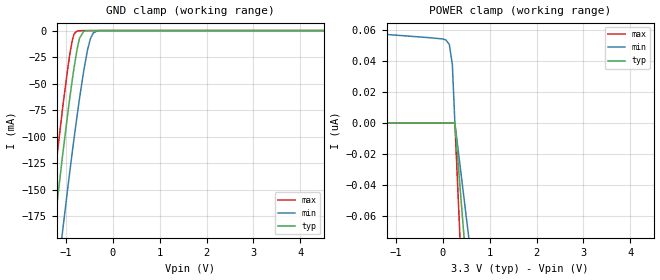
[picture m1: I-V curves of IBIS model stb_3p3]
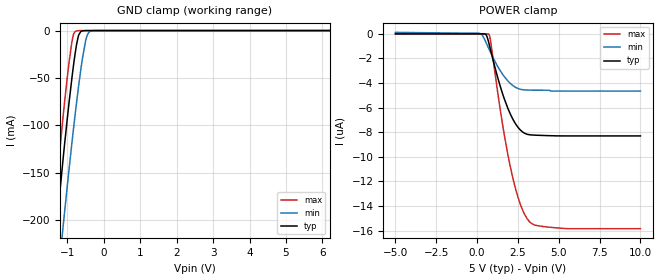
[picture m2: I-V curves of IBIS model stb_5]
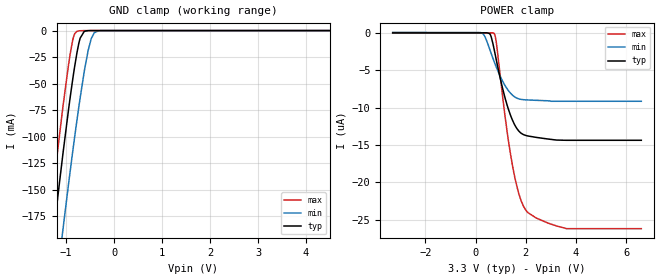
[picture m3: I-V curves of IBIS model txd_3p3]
|Texas Instruments Incorporated
|TCAN1042HGV-Q1 Automotive Fault Protected CAN Transceiver With Flexible
|Data-Rate
|Marketing part#   Digital Voltage Range   Package-type   #pins
|TCAN1042HGVDQ1   3-5.5V   SOIC   8
|TCAN1042HGVDRQ1   3-5.5V   SOIC   8
[IBIS Ver]   4.1
[File name]   tcan1042hgv_q1.ibs
[File Rev]   1.1
[Date]   4/13/2016
[Source]
| Texas Instruments Incorporated.
| Analog-eLab Design Center, HPA
| 12500 TI Blvd
| Dallas, TX -75243
[Notes]   Revision History:
| Rev 1.1: 04/13/2016
| -Second version of the model. Fine tuning canh_os and canl_od models.
| Rev 1.0: 3/31/2016
| - Initial version of the model
| - Model generated from simulations in SPECTRE
| - Model matched to SPICE simulation
| - C_comp although listed in numerical order of value are
|   obtained from varying PVT conditions. For PVT conditions for
|   each specific value refer the buffer description under
|   respective [Model]. IBIS model user is responsible for using
|   appropriate C_comp to simulate for Signal Integrity.
|* EXCEPTION:   *
|* - For models rxd_* pullup and pulldown IV tables does not pass through *
|*   zero because of resistors R6, R8, R14 connected to pad.   *
|* - For canh_os model pullup table does not pass through zero due to   *
|*   resistor network connected to PAD. Power clamp table has leakage due *
|*   to resistor network connected to PAD   *
|* - For canl_od model pulldown table does not pass through zero due to   *
|*   resistor network connected to PAD. Power clamp table has leakage due *
|*   to resistor network connected to PAD   *
|* - canh_os and canl_od VT irregularity not indicitive of silicon   *
|*   actual device shows smooth transition between dominant and recessive *
[Disclaimer]
| This model is designed as an aid for customers of Texas Instruments.
| TI and its licensors and suppliers make no warranties, either expressed
| or implied, with respect to this  model, including the warranties of
| merchantability or fitness for a particular purpose. The model is
| provided solely on an "as is" basis. The entire risk as to its quality
| and performance is with the customer.
[Copyright]
(C) Copyright 2016 Texas Instruments Incorporated.All rights reserved.
|   TCAN1042HGV_Q1D
[Component]   TCAN1042HGV_Q1D
[Manufacturer]   TI
[Package]   |8 SOIC - D Package
|   typ   min   max
R_pkg   0.068   0.038   0.098
L_pkg   2.235nH   1.713nH   2.756nH
C_pkg   0.393pF   0.337pF   0.449pF
[Pin]  signal_name   model_name   R_pin   L_pin   C_pin
1   TXD   txd   0.093   2.653n   0.337p
2   GND   gnd   0.038   1.716n   0.449p
3   VCC   power   0.038   1.713n   0.449p
4   RXD   rxd   0.093   2.657n   0.337p
5   VIO   power   0.098   2.756n   0.341p
6   CANL   canl_od   0.092   2.624n   0.363p
7   CANH   canh_os   0.075   2.301n   0.349p
8   STB   stb   0.094   2.677n   0.338p
[Diff_pin]   inv_pin   vdiff   tdelay_typ   tdelay_min   tdelay_max
7   6   NA   NA   NA   NA
|   Model Selectors
[Model Selector] stb
stb_3p3   3.3V   digital Input
stb_5   5.0V   digital Input
[Model Selector] txd
txd_3p3   3.3V   digital Input
txd_5   5.0V   digital Input
[Model Selector] rxd
rxd_3p3   3.3V   digital Output
rxd_5   5.0V   digital Output
| Models and submodels in the file (8): stb_3p3 (Input), stb_5 (Input), txd_3p3 (Input), txd_5 (Input), rxd_3p3 (Output), rxd_5 (Output), canh_os (I/O_open_source), canl_od (I/O_open_drain)
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|   stb_3p3 Model
[Model]   stb_3p3
Model_type   Input
Vinl = 0.99
Vinh = 2.31
|   typ   min   max
|   (nom PVT)   (fast PVT)   (slow PVT)
C_comp   2.287e-12   2.118e-12   2.744e-12
| Where nom  PVT is Nominal Process, 3.3V, 27C
|   Fast PVT is Strong Process,  3.6V, -55C
|   Slow PVT is Weak Process,   3V, 150C
[Voltage Range]   3.3   3   3.6
|Junction Temperature
[Temperature Range]   27   150   -55
[Power Clamp Reference]   3.3   3   3.6
[GND Clamp Reference]   0   0   0
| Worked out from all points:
|   GND clamp passes 1 mA (typ) near -0.62 V on its own axis
[GND Clamp]
|   Voltage   I(typ)   I(min)   I(max)
-3.3V     -1.097A    -1.144A    -1.073A
-1.386V   -241.5mA   -312mA     -198.2mA
-1.234V   -180.4mA   -251.7mA   -136mA
-1.066V   -115.8mA   -187.2mA   -71.51mA
-950.4mV  -74.68mA   -144.9mA   -32.42mA
-866.4mV  -47.18mA   -115.3mA   -9.84mA
-772.2mV  -20.38mA   -83.74mA   -682.4uA
-708mV    -7.173mA   -63.48mA   -166.8uA
-540mV    -73.56uA   -18.53mA   -2.625uA
-475.2mV  -13.82uA   -7.402mA   -445.1nA
-330mV    -246.1nA   -260uA     -18.22nA
6.6V      0A         0A         0A
[POWER Clamp]
|   Voltage   I(typ)   I(min)   I(max)
-3.3V     0A         61.82nA    0A
-330mV    0A         55.05nA    0A
-3mV      0A         54.15nA    0A
-2.4mV    0A         54.14nA    0A
0V        0A         54.13nA    0A
1.2mV     0A         54.12nA    0A
3mV       0A         54.11nA    0A
66mV      0A         53.48nA    0A
138mV     0A         50.7nA     0A
204mV     0A         37.79nA    0A
258mV     0A         0A         0A
6.6V      -2.384uA   -1.58uA    -4.306uA
|   stb_5 Model
[Model]   stb_5
Model_type   Input
Vinl = 1.5
Vinh = 3.5
|   typ   min   max
|   (nom PVT)   (fast PVT)   (slow PVT)
C_comp   2.287e-12   2.118e-12   2.744e-12
| Where nom  PVT is Nominal Process, 5V, 27C
|   Fast PVT is Strong Process,  5.5V, -55C
|   Slow PVT is Weak Process,   4.5V, 150C
[Voltage Range]   5   4.5   5.5
|Junction Temperature
[Temperature Range]   27   150   -55
[Power Clamp Reference]   5   4.5   5.5
[GND Clamp Reference]   0   0   0
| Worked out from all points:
|   GND clamp passes 1 mA (typ) near -0.63 V on its own axis
[GND Clamp]
|   Voltage   I(typ)   I(min)   I(max)
-5V       -1.891A    -1.922A    -1.879A
-1.522V   -297.1mA   -366.4mA   -255mA
-1.373V   -235.5mA   -306.2mA   -192mA
-1.115V   -133.6mA   -205.2mA   -88.9mA
-960mV    -77.39mA   -147.8mA   -34.81mA
-875mV    -49.33mA   -117.7mA   -11.28mA
-825.5mV  -34.35mA   -100.8mA   -3.153mA
-750mV    -14.76mA   -76.12mA   -386.7uA
-630mV    -838.1uA   -40.3mA    -25.63uA
-500mV    -25uA      -10.78mA   -774.5nA
-329mV    -233.3nA   -243.6uA   -34.68nA
10V       0A         0A         0A
[POWER Clamp]
|   Voltage   I(typ)   I(min)   I(max)
-5V       0A         120.9nA    0A
152.5mV   0A         51.48nA    0A
530.5mV   -35.11nA   -651.8nA   0A
725.5mV   -775.6nA   -1.229uA   -37.31nA
863mV     -1.51uA    -1.624uA   -924.4nA
1.6V      -5.031uA   -3.361uA   -7.707uA
2.11V     -6.734uA   -4.12uA    -11.27uA
2.407V    -7.425uA   -4.386uA   -12.86uA
2.772V    -7.967uA   -4.541uA   -14.29uA
3.344V    -8.225uA   -4.576uA   -15.43uA
5.505V    -8.303uA   -4.653uA   -15.85uA
10V       -8.303uA   -4.653uA   -15.85uA
|   txd_3p3 Model
[Model]   txd_3p3
Model_type   Input
Vinl = 0.99
Vinh = 2.31
|   typ   min   max
|   (nom PVT)   (fast PVT)   (slow PVT)
C_comp   2.287e-12   2.118e-12   2.744e-12
| Where nom  PVT is Nominal Process, 3.3V, 27C
|   Fast PVT is Strong Process,  3.6V, -55C
|   Slow PVT is Weak Process,   3V, 150C
[Voltage Range]   3.3   3   3.6
|Junction Temperature
[Temperature Range]   27   150   -55
[Power Clamp Reference]   3.3   3   3.6
[GND Clamp Reference]   0   0   0
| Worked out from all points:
|   GND clamp passes 1 mA (typ) near -0.62 V on its own axis
[GND Clamp]
|   Voltage   I(typ)   I(min)   I(max)
-3.3V     -1.097A    -1.144A    -1.073A
-1.386V   -241.5mA   -312mA     -198.2mA
-1.234V   -180.4mA   -251.7mA   -136mA
-1.066V   -115.8mA   -187.2mA   -71.49mA
-950.4mV  -74.68mA   -144.8mA   -32.4mA
-866.4mV  -47.17mA   -115.3mA   -9.833mA
-772.2mV  -20.38mA   -83.73mA   -677.4uA
-708mV    -7.169mA   -63.47mA   -163.5uA
-540mV    -73.3uA    -18.53mA   -2.704uA
-475.2mV  -13.88uA   -7.4mA     -723.7nA
-330mV    -361.7nA   -259.8uA   -278.1nA
6.6V      0A         0A         0A
[POWER Clamp]
|   Voltage   I(typ)   I(min)   I(max)
-3.3V     0A         61.83nA    0A
198mV     0A         38.13nA    0A
375mV     0A         -528.7nA   0A
558mV     -98.16nA   -2.148uA   0A
735.6mV   -2.148uA   -3.81uA    -62.66nA
831mV     -3.708uA   -4.639uA   -1.439uA
1.179V    -8.775uA   -7.084uA   -11.3uA
1.449V    -11.53uA   -8.275uA   -17.37uA
1.722V    -13.15uA   -8.838uA   -21.53uA
1.996V    -13.73uA   -8.968uA   -23.71uA
3.623V    -14.38uA   -9.159uA   -26.21uA
6.6V      -14.38uA   -9.159uA   -26.21uA
